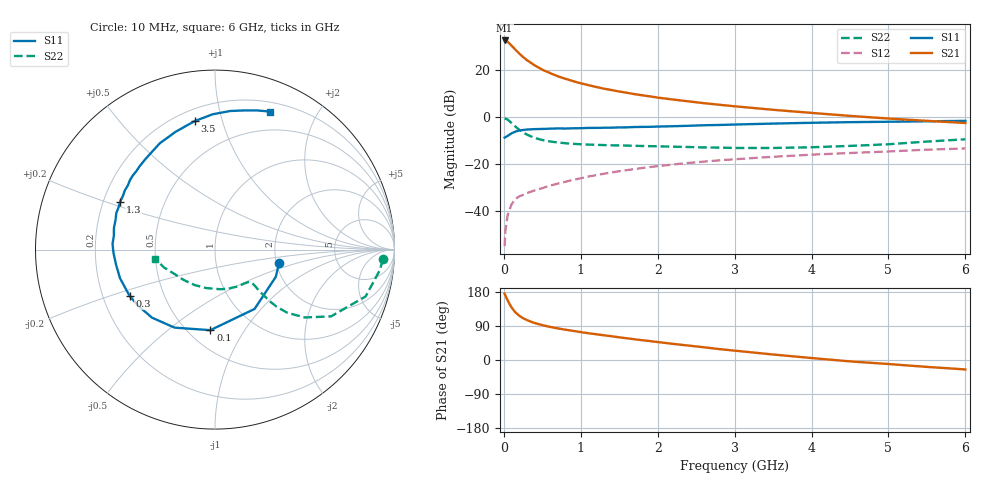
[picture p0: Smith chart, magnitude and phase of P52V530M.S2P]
! SIEMENS Small Signal Semiconductors
! BFP183
! Si NPN RF Bipolar Junction Transistor in SOT143
! VCE = 2.5 V  IC = 30 mA
! Common Emitter S-Parameters:  March  1996
# GHz  S  MA  R  50
!  f  S11  S21  S12  S22
! GHz  MAG  ANG  MAG  ANG  MAG  ANG  MAG  ANG
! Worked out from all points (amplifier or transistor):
!   36 points, 10 MHz to 6 GHz, reference 50 ohm
!   highest |S21| = 32.5 dB at 10 MHz (marker M1)
!   |S21| within 3 dB of that: start of sweep to 123.8 MHz
!   unconditionally stable (mu >= 1): 575.2 MHz to 5.717 GHz
!   at 250 MHz: K = 0.64, MSG = 29.3 dB, |S12| = -33.1 dB
!   at 1.4 GHz: K = 1.21, MAG = 14.8 dB, |S12| = -23.6 dB
!   at 6 GHz: K = 0.98, MSG = 5.4 dB, |S12| = -13.4 dB
!   S11 on the Smith chart (normalised r, x): 10 MHz: 2.07, -0.36; 100 MHz: 0.64, -0.72; 300 MHz: 0.31, -0.23; 1.3 GHz: 0.27, +0.22; 3.5 GHz: 0.27, +0.82; 6 GHz: 0.29, +1.44
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0.01  0.3648 -12.1  42.33 175.1  0.0018 73.3  0.9373 -3.3
0.02  0.3711 -24.2  42.18 170.5  0.0038 87.2  0.9256 -7.1
0.05  0.3974 -56.3  39.73 156.7  0.0083 73.4  0.8787 -17.3
0.1  0.4496 -93.3  32.95 138.7  0.014 60.8  0.7462 -29.9
0.15  0.4897 -117.4  26.99 125.8  0.0181 54.7  0.6268 -37.1
0.2  0.5168 -132.8  22.36 116.9  0.0206 51.7  0.5358 -41.1
0.25  0.5296 -143.4  18.82 110.3  0.0221 51.1  0.4706 -42.8
0.3  0.5413 -151.6  16.18 105.4  0.0242 50.6  0.4221 -43.3
0.4  0.5529 -163.3  12.55 97.6  0.0275 52.1  0.3603 -43.2
0.5  0.5578 -171.4  10.14 92.1  0.0308 52.8  0.3243 -42.8
0.6  0.5656 -178.0  8.592 87.4  0.0348 54.8  0.3022 -42.3
0.7  0.5718 176.9  7.347 83.5  0.0384 56.4  0.2873 -42.1
0.8  0.5688 172.2  6.49 80.0  0.042 56.9  0.2772 -42.3
1.1  0.5865 159.6  4.752 70.6  0.0544 57.4  0.2589 -44.4
1.3  0.5918 153.2  4.005 65.2  0.0623 57.2  0.2532 -47.1
1.7  0.6125 140.5  3.058 54.7  0.0783 55.3  0.2444 -53.8
2.2  0.6368 127.2  2.349 42.5  0.098 51.4  0.2338 -64.6
2.8  0.6779 112.8  1.822 28.8  0.1199 45.7  0.2237 -80.9
3.5  0.7248 99.0  1.422 14.5  0.1428 39.4  0.2198 -102.8
4.5  0.777 83.7  1.056 -3.7  0.1718 29.9  0.2431 -135.8
5.5  0.8103 73.1  0.829 -18.2  0.2024 21.7  0.3007 -160.6
6  0.8279 68.2  0.746 -24.9  0.2148 16.9  0.3361 -171.2
